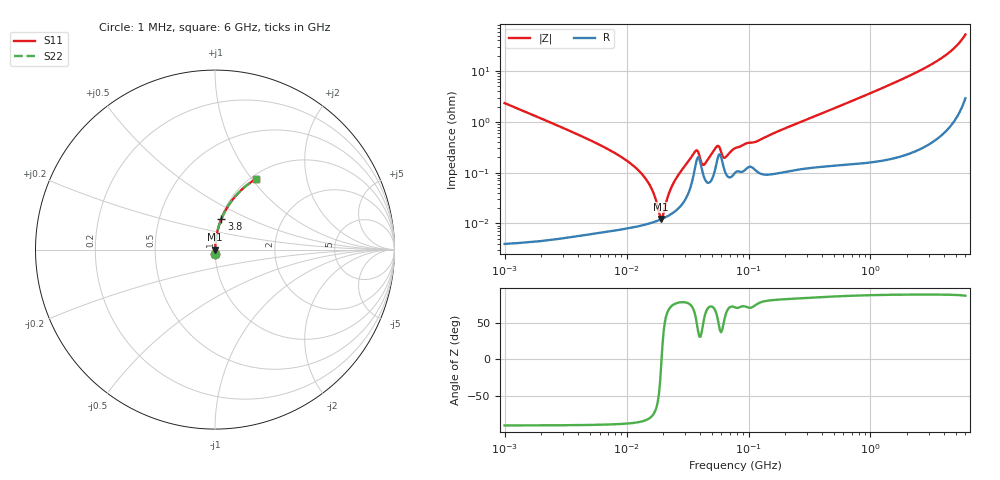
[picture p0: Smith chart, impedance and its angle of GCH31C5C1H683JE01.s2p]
!Murata Part Number: GCH31C5C1H683JE01
!These Parameters are Measured in Series Mode Connection
!Data Generated on Mar 13, 2026
!  o--ll--o
!Port1  Port2
!  o------o
!Operation Temp=25[degC], DC Bias Voltage=0[V]
!Freq. Start=1000[kHz] Stop=6[GHz] 401[Steps]
# Hz S RI R 50
!Freq.(Hz) S11(Real) S11(Imag) S21(Real) S21(Imag) S12(Real) S12(Imag) S22(Real) S22(Imag)
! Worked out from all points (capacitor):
!   401 points, 1 MHz to 6 GHz, reference 50 ohm
!   read as one part in series: C = 67.9 nF near 1.044 MHz
!   lowest |Z| = 12.2 mohm at 19.26 MHz (marker M1)
!   series resonance near 19.36 MHz, so ESL is about 1 nH
!   S11 on the Smith chart (normalised r, x): 1 MHz: 1.00, -0.05; 3.8 GHz: 1.01, +0.36; 6 GHz: 1.06, +1.05
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1000000  0.000586 -0.0234  0.9994 0.0234  0.9994 0.0234  0.000586 -0.0234
4293785  8.46e-05 -0.00519  0.9999 0.00519  0.9999 0.00519  8.46e-05 -0.00519
8426497  7.88e-05 -0.00226  0.9999 0.00226  0.9999 0.00226  7.88e-05 -0.00226
1.246418e7  8.89e-05 -0.00112  0.9999 0.00112  0.9999 0.00112  8.89e-05 -0.00112
1.583299e7  0.000102 -0.000503  0.9999 0.000503  0.9999 0.000503  0.000102 -0.000503
1.843659e7  0.000116 -0.000123  0.9999 0.000123  0.9999 0.000123  0.000116 -0.000123
1.925624e7  0.000121 -1.34e-05  0.9999 1.34e-05  0.9999 1.34e-05  0.000121 -1.34e-05
2.011232e7  0.000127 9.73e-05  0.9999 -9.73e-05  0.9999 -9.73e-05  0.000127 9.73e-05
2.194036e7  0.000141 0.000324  0.9999 -0.000324  0.9999 -0.000324  0.000141 0.000324
2.44608e7  0.000167 0.000625  0.9998 -0.000625  0.9998 -0.000625  0.000167 0.000625
3.618157e7  0.00115 0.00226  0.9989 -0.00226  0.9989 -0.00226  0.00115 0.00226
3.779011e7  0.00185 0.00203  0.9982 -0.00203  0.9982 -0.00203  0.00185 0.00203
4.305766e7  0.00083 0.00115  0.9992 -0.00115  0.9992 -0.00115  0.00083 0.00115
5.469524e7  0.00154 0.00284  0.9985 -0.00284  0.9985 -0.00284  0.00154 0.00284
5.712686e7  0.00227 0.00241  0.9977 -0.00241  0.9977 -0.00241  0.00227 0.00241
6.368941e7  0.0011 0.00161  0.9989 -0.00161  0.9989 -0.00161  0.0011 0.00161
7.745967e7  0.000996 0.00286  0.999 -0.00286  0.999 -0.00286  0.000996 0.00286
3.325952e8  0.00139 0.0122  0.9986 -0.0122  0.9986 -0.0122  0.00139 0.0122
1.428092e9  0.00463 0.0529  0.9954 -0.0529  0.9954 -0.0529  0.00463 0.0529
3.800129e9  0.0356 0.1708  0.9644 -0.1708  0.9644 -0.1708  0.0356 0.1708
4.93336e9  0.0874 0.2645  0.9126 -0.2645  0.9126 -0.2645  0.0874 0.2645
6e9  0.2286 0.3932  0.7714 -0.3932  0.7714 -0.3932  0.2286 0.3932
